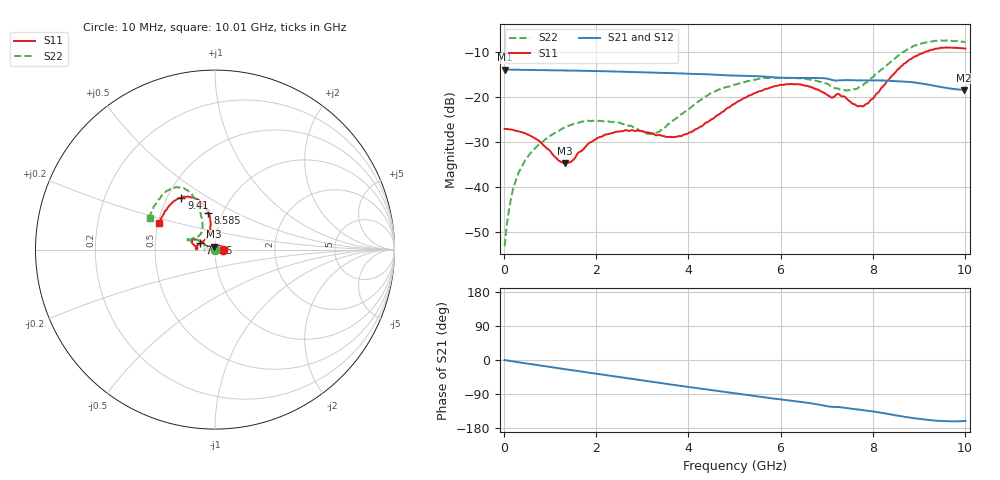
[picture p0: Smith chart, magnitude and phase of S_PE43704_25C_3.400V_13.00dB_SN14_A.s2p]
! Device ID: PE43704
! Dir: z:\PE43704\PE43704_Char_1_20130516\PE43704\AMB\3p400V\13p00dB
! Serial: 14
! Insertion: A
! Impedance: 50 ohm
! Temp: Amb
! VDD: 3.400V
! Attenuation Step: 13.00dB
! IDD: 1.139585e-01mA
#  Hz  S  RI  R  50
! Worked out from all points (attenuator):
!   401 points, 10 MHz to 10.01 GHz, reference 50 ohm
!   highest |S21| = -13.94 dB at 10 MHz (marker M1); lowest = -18.5 dB at 9.985 GHz (marker M2)
!   lowest |S11| = -34.8 dB at 1.31 GHz (marker M3), VSWR 1.04, Z = 49.2 + j1.62 ohm
!   |S11| at or under -10 dB: start of sweep to 9.141 GHz
!   |S22| runs from -53.3 to -7.5 dB; largest |S21 - S12| = 0.0015
!   S11 on the Smith chart (normalised r, x): 10 MHz: 1.09, +0.00; 7.485 GHz: 0.84, +0.06; 8.585 GHz: 0.85, +0.37; 9.41 GHz: 0.59, +0.39; 10.01 GHz: 0.51, +0.17
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1e7  0.0437 0.000314  0.2009 -0.000693  0.2009 -0.000609  0.00212 0.000449
1.85e8  0.0422 0.00744  0.1999 -0.0124  0.1999 -0.0124  0.00164 0.00892
4.1e8  0.0367 0.0155  0.1974 -0.0273  0.1975 -0.0267  -0.00268 0.0175
7.35e8  0.0235 0.0231  0.193 -0.0469  0.1929 -0.0468  -0.0143 0.025
1.31e9  -0.00805 0.0164  0.1793 -0.08  0.1794 -0.08  -0.0414 0.0183
1.685e9  -0.0249 0.00291  0.1674 -0.0997  0.1675 -0.0995  -0.0527 0.00513
2.01e9  -0.0331 -0.00894  0.1553 -0.115  0.1553 -0.1149  -0.0534 -0.00541
2.435e9  -0.035 -0.0209  0.1373 -0.1328  0.1374 -0.1328  -0.0501 -0.0116
3.11e9  -0.0322 -0.0241  0.105 -0.1549  0.1052 -0.1547  -0.0388 -0.00193
3.36e9  -0.0321 -0.0196  0.092 -0.1609  0.0923 -0.1608  -0.0402 0.00614
4.01e9  -0.0397 0.00311  0.0576 -0.171  0.0578 -0.171  -0.0667 0.0299
4.46e9  -0.05 0.0206  0.0337 -0.1744  0.0339 -0.1743  -0.0944 0.0524
5.01e9  -0.0733 0.0413  0.00609 -0.172  0.00629 -0.172  -0.1257 0.0535
5.96e9  -0.1217 0.0563  -0.0374 -0.1593  -0.0369 -0.1594  -0.1537 0.0507
6.685e9  -0.1236 0.0312  -0.0683 -0.1471  -0.0683 -0.1469  -0.1453 0.0512
7.485e9  -0.0833 0.0353  -0.0936 -0.1213  -0.0937 -0.1213  -0.0847 0.0834
7.835e9  -0.0462 0.0679  -0.104 -0.1111  -0.104 -0.1114  -0.0704 0.1235
8.36e9  -0.0253 0.1563  -0.1203 -0.0908  -0.1198 -0.091  -0.0859 0.2214
8.585e9  -0.0397 0.2052  -0.1255 -0.0793  -0.1247 -0.0796  -0.1078 0.2724
9.41e9  -0.187 0.2883  -0.1229 -0.0435  -0.123 -0.0429  -0.2571 0.3318
9.985e9  -0.3045 0.1593  -0.1126 -0.0387  -0.1132 -0.0384  -0.3611 0.1857
1.001e10  -0.3098 0.1495  -0.1127 -0.0391  -0.1134 -0.0396  -0.3648 0.177
